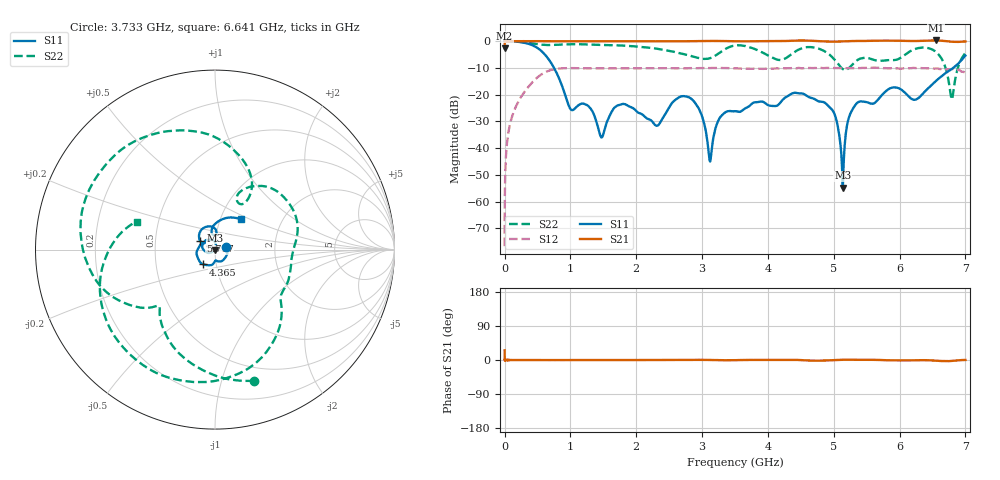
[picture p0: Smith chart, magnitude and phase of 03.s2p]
!Keysight Technologies,N5232A,MY52221221,A.10.65.11
!Date: Wednesday, October 16, 2024 11:51:45
!Correction: S11(Full 2 Port(1,4))
!S41(Full 2 Port(1,4))
!S14(Full 2 Port(1,4))
!S44(Full 2 Port(1,4))
!S2P File: Measurements: S11, S41, S14, S44:
# Hz S  RI  R 50
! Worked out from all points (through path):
!   4001 points, 300 kHz to 7 GHz, reference 50 ohm
!   highest |S21| = 0.26 dB at 6.554 GHz (marker M1); lowest = -2.6 dB at 300 kHz (marker M2)
!   lowest |S11| = -54.8 dB at 5.138 GHz (marker M3), VSWR 1.00, Z = 50.1 - j0.134 ohm
!   |S11| at or under -10 dB: 750.9 MHz to 6.814 GHz (6.063 GHz wide, 160 % of centre)
!   |S22| runs from -21.8 to 0.0 dB; largest |S21 - S12| = 1.3
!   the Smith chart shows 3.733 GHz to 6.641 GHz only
!   S11 on the Smith chart (normalised r, x): 3.733 GHz: 1.13, +0.04; 4.365 GHz: 0.87, -0.14; 5.717 GHz: 0.85, +0.08; 6.641 GHz: 1.25, +0.44
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300000  -0.9915 -0.0163  0.6655 0.3169  0.000147 9.1e-06  -0.9889 -0.0251
7.554678e7  -0.8006 0.5938  0.9974 -0.00625  0.0129 0.0223  -0.9651 0.2447
3.415354e8  0.8927 0.1658  0.9993 -0.000869  0.0872 -0.098  -0.4294 0.8307
4.867792e8  0.281 -0.7091  0.9996 -0.0028  -0.0807 -0.1875  -0.0484 0.8793
6.320229e8  -0.4591 -0.2583  0.9982 -0.00282  -0.2682 0.0109  0.273 0.8045
1.1675e9  0.0312 0.0604  0.9961 -0.00206  0.1648 -0.2643  0.8452 -0.221
1.687228e9  0.0599 0.000827  0.9952 -0.0015  -0.0314 0.3087  -0.133 -0.8276
2.3347e9  -0.00206 0.0269  0.9944 0.000261  -0.2847 -0.1282  -0.6354 0.3265
2.812429e9  0.0771 -0.0417  0.9983 0.00589  0.2947 0.1061  0.1129 0.5244
3.122166e9  0.00204 -0.00526  1.008 0.00231  -0.0519 -0.31  0.3171 0.3609
3.50015e9  -0.0482 0.00903  0.9934 -0.00703  -0.1241 0.2845  0.7896 -0.256
3.73289e9  0.0613 0.0173  0.9947 0.0042  0.2753 0.1271  0.2188 -0.7308
4.364613e9  -0.0653 -0.0825  1.018 0.0106  -0.2521 0.1874  -0.4891 -0.3034
4.66735e9  -0.0824 0.0265  1.016 -0.0282  0.2801 0.1381  -0.6099 0.4712
5.13808e9  0.00123 -0.00134  0.989 0.00933  -0.2868 -0.1271  0.1577 0.2552
5.292073e9  -0.0539 -0.0104  1.004 0.0103  -0.2543 0.1821  0.1616 0.3369
5.717305e9  -0.0814 0.0466  1.027 -0.00108  0.2931 -0.122  0.4257 -0.0597
5.83455e9  -0.0858 0.0939  1.024 -0.0122  0.1147 -0.2875  0.4082 -0.1725
6.553769e9  0.0517 0.1731  1.03 -0.0321  0.3075 0.0228  -0.6221 -0.0801
6.641265e9  0.1433 0.1694  1.017 -0.0485  0.2596 -0.1597  -0.4368 0.1562
6.795259e9  0.2904 -0.0884  0.9757 -0.0418  -0.0391 -0.2982  -0.0813 -0.00707
7e9  -0.4442 -0.302  0.9888 0.00141  -0.2481 0.053  -0.5979 -0.039
